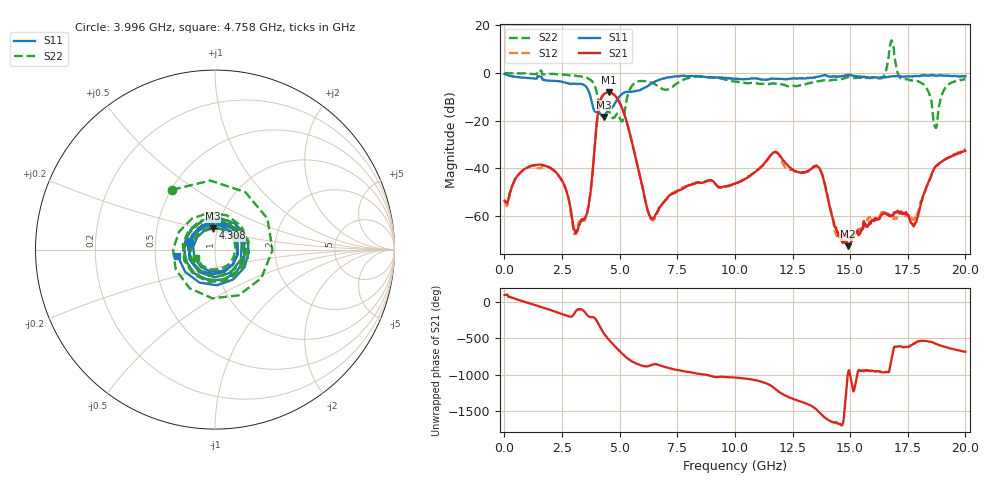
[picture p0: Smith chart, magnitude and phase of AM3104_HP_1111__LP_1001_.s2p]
!Created with skrf (http://scikit-rf.org).
# Hz S RI R 50.0
!freq ReS11 ImS11 ReS21 ImS21 ReS12 ImS12 ReS22 ImS22
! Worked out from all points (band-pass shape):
!   1601 points, 10 MHz to 20 GHz, reference 50 ohm
!   highest |S21| = -8.11 dB at 4.52 GHz (marker M1); lowest = -72.8 dB at 14.9 GHz (marker M2)
!   |S21| within 3 dB of the highest: 4.18 GHz to 4.919 GHz (739.1 MHz wide, 16.2 % of centre)
!   lowest |S11| = -18.4 dB at 4.308 GHz (marker M3), VSWR 1.27, Z = 47.4 + j11.4 ohm
!   |S11| at or under -10 dB: 3.737 GHz to 4.976 GHz (1.239 GHz wide, 28.4 % of centre)
!   |S22| runs from -23.1 to 13.7 dB; largest |S21 - S12| = 0.03
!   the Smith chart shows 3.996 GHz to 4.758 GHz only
!   S11 on the Smith chart (normalised r, x): 3.996 GHz: 0.74, +0.06; 4.308 GHz: 0.95, +0.23; 4.758 GHz: 0.65, -0.05
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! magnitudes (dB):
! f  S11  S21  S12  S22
! 10 MHz  -0.4  -53.6  -53.9  -0.1
! 1.759 GHz  -3.0  -39.0  -39.1  -0.6
! 2.559 GHz  -3.8  -46.2  -46.3  -0.7
! 3.058 GHz  -4.5  -66.2  -67.6  -1.1
! 3.346 GHz  -4.6  -61.7  -61.4  -1.5
! 3.658 GHz  -7.7  -55.5  -55.9  -2.4
! 3.996 GHz  -16.3  -22.3  -22.4  -7.8
! 4.308 GHz  -18.4  -9.0  -9.0  -14.9
! 4.52 GHz  -15.4  -8.1  -8.2  -16.1
! 4.758 GHz  -13.5  -9.2  -9.2  -18.8
! 6.282 GHz  -5.0  -59.4  -59.8  -4.0
! 6.682 GHz  -3.0  -57.7  -57.3  -5.6
! 10.01 GHz  -2.5  -46.6  -46.6  -3.7
! 11.72 GHz  -2.4  -33.3  -33.3  -4.4
! 13.34 GHz  -2.1  -40.1  -40.0  -4.0
! 14.9 GHz  -0.9  -72.8  -69.6  -1.8
! 16.38 GHz  -1.8  -59.5  -58.6  -2.1
! 16.68 GHz  -1.6  -59.8  -59.7  7.3
! 17.79 GHz  -1.3  -63.6  -61.4  -3.1
! 18.69 GHz  -1.1  -39.4  -39.5  -22.7
! 19.13 GHz  -1.2  -36.3  -36.2  -6.3
! 20 GHz  -1.3  -32.7  -32.1  -2.6
